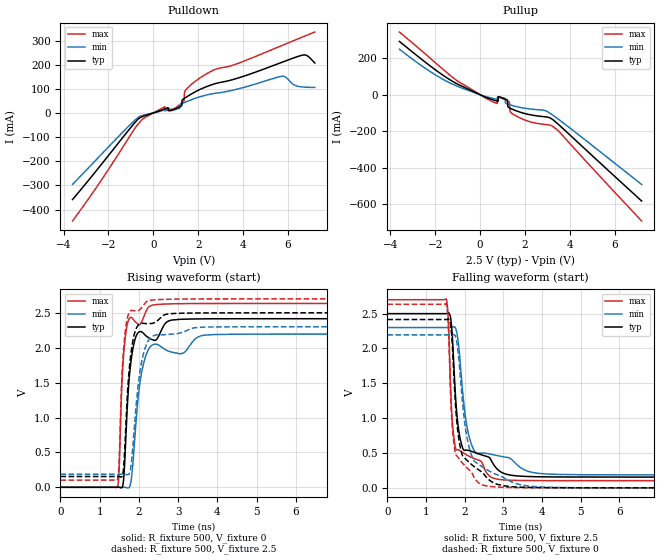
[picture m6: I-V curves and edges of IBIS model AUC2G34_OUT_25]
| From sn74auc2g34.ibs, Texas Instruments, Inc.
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[Model]   AUC2G34_OUT_25
Model_type  Output
Vref =   0
Rref =   500
Cref =   30p
Vmeas =   1.25
| variable   typ   min   max
C_comp   7.47pF   0.23pF   23.67pF
| C_pullup   8.37pF   0.23pF   23.67pF
| C_pulldown   6.58pF   2.12pF   15.80pF
[Temperature Range]   40   100   -40
| Ambient temperature   25   85   -40
[Voltage range]   2.5   2.3   2.7
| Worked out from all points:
|   slope of the pulldown table from 0 to 0.375 V, typ, clamps not added: 30.9 ohm
|   slope of the pullup table from 0 to 0.375 V, typ, clamps not added: 19.2 ohm
|   rising waveform, R_fixture 500, V_fixture 0: 20-80 % time 183ps typ, 252ps min, 132ps max; typ from 0 V to 2.42 V
|   falling waveform, R_fixture 500, V_fixture 2.5: 20-80 % time 224ps typ, 313ps min, 153ps max; typ from 2.5 V to 0.154 V
|   rising waveform, R_fixture 500, V_fixture 2.5: 20-80 % time 180ps typ, 250ps min, 130ps max; typ from 0.154 V to 2.5 V
|   falling waveform, R_fixture 500, V_fixture 0: 20-80 % time 237ps typ, 334ps min, 156ps max; typ from 2.42 V to 0 V
[Pulldown]
| AUC2G34_OUT_25
|   Voltage   I(typ)   I(min)   I(max)
-3.6V     -358.4mA   -295.5mA   -447.3mA
-445mV    -13.39mA   -9.086mA   -23.04mA
515mV     17.02mA    12.57mA    25.99mA
1.025V    18.9mA     15.4mA     23.61mA
1.27V     30.1mA     38.43mA    41.47mA
1.37V     59.42mA    42.49mA    49.07mA
1.395V    60.94mA    43.5mA     85.27mA
1.48V     66.06mA    46.86mA    98.94mA
2.545V    115mA      77.99mA    170.9mA
5.695V    208.5mA    151.5mA    277.9mA
6.74V     240.5mA    107.2mA    317.9mA
7.2V      207mA      105.9mA    335.2mA
[Pullup]
| AUC2G34_OUT_25
|   Voltage   I(typ)   I(min)   I(max)
-3.6V     292.7mA    249.8mA    344.4mA
-960mV    55.5mA     44.14mA    71.52mA
730mV     -33.82mA   -24.42mA   -47.21mA
760mV     -34.84mA   -25.13mA   -47.16mA
770mV     -35.18mA   -25.36mA   -13.07mA
1.115V    -23.95mA   -20.34mA   -27.78mA
1.215V    -28.93mA   -50.57mA   -34.8mA
1.295V    -71.17mA   -53.86mA   -40.35mA
1.345V    -74.43mA   -55.82mA   -93.46mA
1.755V    -94.55mA   -68.88mA   -126.2mA
3.305V    -143.1mA   -117.6mA   -180mA
7.2V      -583.3mA   -492.5mA   -693.2mA
[Ramp]
| AUC2G34_OUT_25
| variable   typ   min   max
dV/dt_r   1.45/1.84E-10   1.32/2.52E-10   1.58/1.33E-10
dV/dt_f   1.41/2.24E-10   1.27/3.14E-10   1.57/1.53E-10
R_load = 500
[Rising Waveform]
| AUC2G34_OUT_25
R_fixture =   500
C_fixture =   0
L_fixture =   0
V_fixture =   0
V_fixture_min = 0
V_fixture_max = 0
|   Time   V(typ)   V(min)   V(max)
0s        9.76nV     28.57nV    1.856nV
1.46ns    597.8uV    52.8uV     14.99mV
1.6ns     62.72mV    1.113mV    1.819V
1.695ns   1.053V     -7.115mV   2.311V
1.8ns     1.813V     94.45mV    2.435V
1.915ns   2.146V     859.8mV    2.367V
2.085ns   2.222V     1.691V     2.388V
2.355ns   2.112V     2.044V     2.611V
3.18ns    2.409V     1.944V     2.632V
22ns      2.416V     2.195V     2.634V
[Falling Waveform]
| AUC2G34_OUT_25
R_fixture =   500
C_fixture =   0
L_fixture =   0
V_fixture =   2.5
V_fixture_min = 2.3
V_fixture_max = 2.7
|   Time   V(typ)   V(min)   V(max)
0s        2.5V       2.3V       2.7V
1.525ns   2.5V       2.3V       2.712V
1.58ns    2.511V     2.3V       2.375V
1.65ns    2.381V     2.303V     1.248V
1.765ns   1.302V     2.289V     569.5mV
1.925ns   612mV      1.527V     516.1mV
2.16ns    527.2mV    648.3mV    441.8mV
2.825ns   278.1mV    465.2mV    126.3mV
4.395ns   156.2mV    193.2mV    103.2mV
22ns      154.5mV    186.3mV    102.6mV
[Rising Waveform]
| AUC2G34_OUT_25
R_fixture =   500
C_fixture =   0
L_fixture =   0
V_fixture =   2.5
V_fixture_min = 2.3
V_fixture_max = 2.7
|   Time   V(typ)   V(min)   V(max)
0s        154.5mV    186.3mV    102.6mV
1.46ns    155mV      186.3mV    118.9mV
1.495ns   155mV      186.4mV    368.3mV
1.6ns     229.3mV    187.3mV    1.91V
1.685ns   1.108V     180.5mV    2.37V
1.79ns    1.887V     271.2mV    2.529V
1.88ns    2.19V      830.9mV    2.53V
2.04ns    2.345V     1.706V     2.555V
2.26ns    2.346V     2.119V     2.677V
22ns      2.5V       2.3V       2.7V
[Falling Waveform]
| AUC2G34_OUT_25
R_fixture =   500
C_fixture =   0
L_fixture =   0
V_fixture =   0
V_fixture_min = 0
V_fixture_max = 0
|   Time   V(typ)   V(min)   V(max)
0s        2.416V     2.195V     2.634V
1.525ns   2.415V     2.195V     2.643V
1.575ns   2.422V     2.195V     2.346V
1.645ns   2.301V     2.196V     1.219V
1.76ns    1.218V     2.174V     492.8mV
1.895ns   561.5mV    1.542V     387.4mV
2.1ns     374.4mV    617.5mV    265.8mV
2.535ns   170.4mV    273.8mV    31.12mV
4.255ns   1.852mV    7.269mV    517.4uV
22ns      21uV       2.082uV    9.659uV
